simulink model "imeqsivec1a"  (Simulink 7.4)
settings: Solver=ode45  StartTime=0.0  StopTime=1  MaxStep=1e-3  RelTol=1e-3
libraries: simulink x1

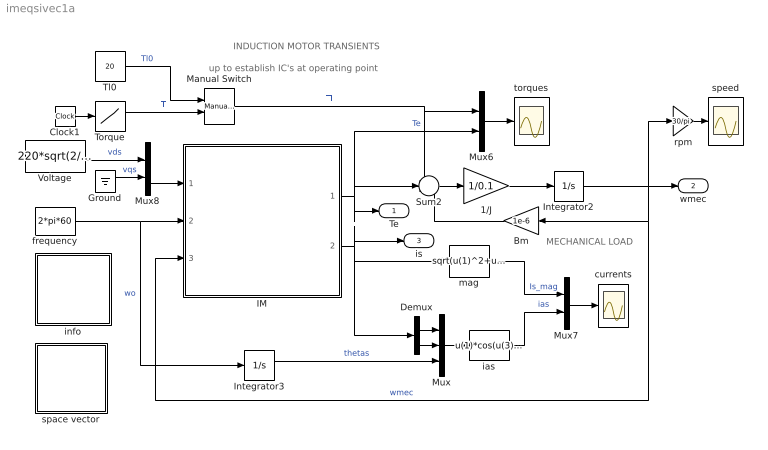
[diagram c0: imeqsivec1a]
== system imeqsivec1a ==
  note: INDUCTION MOTOR TRANSIENTS
  note: MECHANICAL LOAD
  note: up to establish IC's at operating point
  1/J : Gain  Gain=1/0.1  ParameterDataType=sfix(16)  ParameterScaling=2^0  OutDataType=sfix(16)  OutScaling=2^0
  Bm : Gain  Gain=1e-6  ParameterDataType=sfix(16)  ParameterScaling=2^0  OutDataType=sfix(16)  OutScaling=2^0
  Clock1 : Clock
  Demux : Demux  Outputs=2
  Ground : Ground
  IM : Subsystem  mask(Inductionmachine){Rs=0.531, Rr=0.408, Lsl=0.0025, Lrl=0.0025, Lm=0.085, wo=2*pi*60, p=4}
      mask prompts: Rs "Stator resistance [ohm]"; Rr "Rotor resistance [ohm]"; Lsl "Stator leakage inductance  [H]"; Lrl "Rotor leakage inductance [H]"; Lm "Magnetizing inductance [H]"; wo "Base frequency [rad/s]"; p "Number of poles"
      mask help: Space vector model of the induction machine in a general frame k. SI units
  Integrator2 : Integrator  InitialCondition=180
  Integrator3 : Integrator
  Manual Switch : simulink/Signal Routing/Manual Switch  SystemSampleTime=-1  sw=0  action=0  varsize=off
  Mux : Mux  Inputs=3
  Mux6 : Mux  Inputs=2
  Mux7 : Mux  Inputs=2
  Mux8 : Mux  Inputs=2
  Sum2 : Sum  Inputs=-+-  OutDataType=sfix(16)  OutScaling=2^0
  Tl0 : Constant  Value=20  OutDataType=sfix(16)  OutScaling=2^0
  Torque : Lookup  InputValues=[0 0.2 0.2 0.5 0.5 1]  Table=[20 20 10 10 20 20]  OutDataType=sfix(16)  OutScaling=2^0
  Voltage : Constant  Value=220*sqrt(2/3)  OutDataType=sfix(16)  OutScaling=2^0
  currents : Scope
  frequency : Constant  Value=2*pi*60  OutDataType=sfix(16)  OutScaling=2^0
  ias : Fcn  Expr=u(1)*cos(u(3))-u(2)*sin(u(3))
  info : Subsystem
  mag : Fcn  Expr=sqrt(u(1)^2+u(2)^2)
  rpm : Gain  Gain=30/pi  ParameterDataType=sfix(16)  ParameterScaling=2^0  OutDataType=sfix(16)  OutScaling=2^0
  space vector : Subsystem
  speed : Scope
  torques : Scope
  Te : Outport
  wmec : Outport  Port=2
  is : Outport  Port=3
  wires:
  mag/1 -> Mux7/1  "Is_mag"
  Sum2/1 -> 1/J/1
  1/J/1 -> Integrator2/1
  Mux8/1 -> IM/1(vs)
  Ground/1 -> Mux8/2  "vqs"
  IM/1(Te) -> Sum2/2, Te/1, Mux6/2  "Te"
  IM/2(is) -> is/1, Demux/1, mag/1
  Mux6/1 -> torques/1
  Bm/1 -> Sum2/3
  Mux7/1 -> currents/1
  Voltage/1 -> Mux8/1  "vds"
  frequency/1 -> Integrator3/1, IM/2(wk)  "wo"
  Demux/1 -> Mux/1
  Demux/2 -> Mux/2
  Mux/1 -> ias/1
  ias/1 -> Mux7/2  "ias"
  Integrator3/1 -> Mux/3  "thetas"
  Clock1/1 -> Torque/1
  Torque/1 -> Manual Switch/2  "Tl"
  Tl0/1 -> Manual Switch/1  "Tl0"
  Manual Switch/1 -> Mux6/1, Sum2/1  "Tl"
  Integrator2/1 -> wmec/1, IM/3(wmec), Bm/1, rpm/1  "wmec"
  rpm/1 -> speed/1

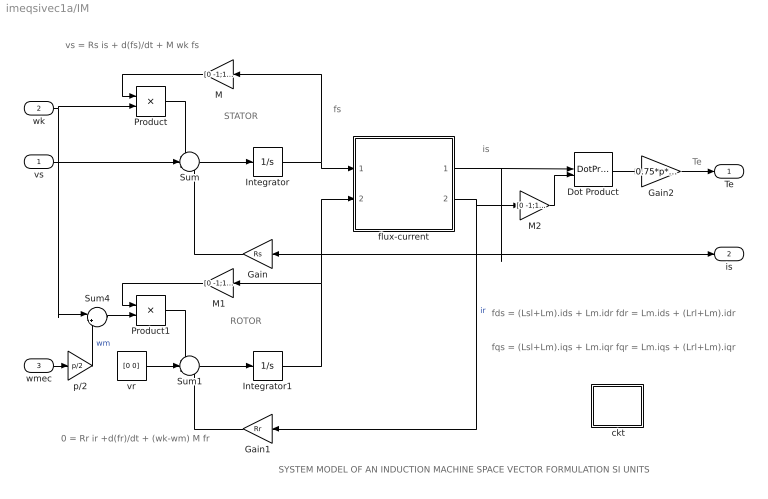
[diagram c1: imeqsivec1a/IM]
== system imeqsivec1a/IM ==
  note: ROTOR
  note: STATOR
  note: fs
  note: is
  note: Te
  note: SYSTEM MODEL OF AN INDUCTION MACHINE SPACE VECTOR FORMULATION SI UNITS
  note: vs = Rs is + d(fs)/dt + M wk fs
  note: 0 = Rr ir +d(fr)/dt + (wk-wm) M fr
  note: fds = (Lsl+Lm).ids + Lm.idr fdr = Lm.ids + (Lrl+Lm).idr
  note: fqs = (Lsl+Lm).iqs + Lm.iqr fqr = Lm.iqs + (Lrl+Lm).iqr
  vs : Inport  OutDataType=sfix(16)  OutScaling=2^0
  wk : Inport  Port=2  OutDataType=sfix(16)  OutScaling=2^0
  wmec : Inport  Port=3  OutDataType=sfix(16)  OutScaling=2^0
  " ckt" : Subsystem
  Dot Product : DotProduct  OutDataType=fixdt(1, 16)  OutScaling=2^-10
  Gain : Gain  Gain=Rs  ParameterDataType=sfix(16)  ParameterScaling=2^0  OutDataType=sfix(16)  OutScaling=2^0
  Gain1 : Gain  Gain=Rr  ParameterDataType=sfix(16)  ParameterScaling=2^0  OutDataType=sfix(16)  OutScaling=2^0
  Gain2 : Gain  Gain=0.75*p*Lm  ParameterDataType=sfix(16)  ParameterScaling=2^0  OutDataType=sfix(16)  OutScaling=2^0
  Integrator : Integrator  InitialCondition=[0 0]
  Integrator1 : Integrator  InitialCondition=[0 0]
  M : Gain  Gain=[0 -1;1 0]  Multiplication=Matrix(K*u)  ParameterDataType=sfix(16)  ParameterScaling=2^0  OutDataType=sfix(16)  OutScaling=2^0
  M1 : Gain  Gain=[0 -1;1 0]  Multiplication=Matrix(K*u)  ParameterDataType=sfix(16)  ParameterScaling=2^0  OutDataType=sfix(16)  OutScaling=2^0
  M2 : Gain  Gain=[0 -1;1 0]  Multiplication=Matrix(K*u)  ParameterDataType=sfix(16)  ParameterScaling=2^0  OutDataType=sfix(16)  OutScaling=2^0
  Product : Product  OutDataType=sfix(16)  OutScaling=2^0
  Product1 : Product  OutDataType=sfix(16)  OutScaling=2^0
  Sum : Sum  Inputs=-+-  OutDataType=sfix(16)  OutScaling=2^0
  Sum1 : Sum  Inputs=-+-  OutDataType=sfix(16)  OutScaling=2^0
  Sum4 : Sum  Inputs=|+-  OutDataType=sfix(16)  OutScaling=2^0
  flux-current : Subsystem
  p/2 : Gain  Gain=p/2  ParameterDataType=sfix(16)  ParameterScaling=2^0  OutDataType=sfix(16)  OutScaling=2^0
  vr : Constant  Value=[0 0]  OutDataType=sfix(16)  OutScaling=2^0
  Te : Outport
  is : Outport  Port=2
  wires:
  Gain/1 -> Sum/3
  vr/1 -> Sum1/2
  Gain1/1 -> Sum1/3
  Integrator/1 -> flux-current/1(fs), M/1
  Integrator1/1 -> flux-current/2(fr), M1/1
  Product1/1 -> Sum1/1
  M1/1 -> Product1/1
  Product/1 -> Sum/1
  M/1 -> Product/1
  Sum4/1 -> Product1/2
  vs/1 -> Sum/2
  wk/1 -> Product/2, Sum4/1
  Sum1/1 -> Integrator1/1
  Sum/1 -> Integrator/1
  flux-current/1(is) -> Gain/1, is/1, Dot Product/1
  flux-current/2(ir) -> Gain1/1, M2/1  "ir"
  Dot Product/1 -> Gain2/1
  Gain2/1 -> Te/1
  wmec/1 -> p/2/1
  p/2/1 -> Sum4/2  "wm"
  M2/1 -> Dot Product/2

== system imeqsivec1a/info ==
  note: Running of an induction motor under balanced sinusoidal excitation
  note: This demonstration illustrates the steady-state running of an induction motor at a specified load followed by sudden step changes in load. First establish the operating point IC's by connecting the manual switch to the up position and saving to workspace the simulation parameters defined as "Final state" ic; Run the simulation for a long enough time to reach a steady-state condition (dc). Then switch down and load from workspace the previously computed ic as "Initial state". Finally rerun the simulation. To modify the machine parameters, double click the induction motor block.

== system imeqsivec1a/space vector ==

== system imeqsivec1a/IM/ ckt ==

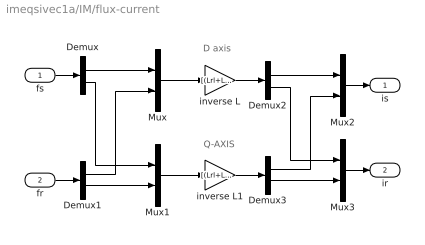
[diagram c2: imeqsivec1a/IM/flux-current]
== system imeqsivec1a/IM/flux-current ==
  note: D axis
  note: Q-AXIS
  fs : Inport  OutDataType=sfix(16)  OutScaling=2^0
  fr : Inport  Port=2  OutDataType=sfix(16)  OutScaling=2^0
  Demux{,1..3} (4 alike) : Demux  Outputs=2
  Mux{,1..3} (4 alike) : Mux  Inputs=2
  inverse L : Gain  Gain=[(Lrl+Lm) -Lm;-Lm (Lsl+Lm)]/(Lsl*Lrl+Lsl*Lm+Lrl*Lm)  Multiplication=Matrix(K*u)  ParameterDataType=sfix(16)  ParameterScaling=2^0  OutDataType=sfix(16)  OutScaling=2^0
  inverse L1 : Gain  Gain=[(Lrl+Lm) -Lm;-Lm (Lsl+Lm)]/(Lsl*Lrl+Lsl*Lm+Lrl*Lm)  Multiplication=Matrix(K*u)  ParameterDataType=sfix(16)  ParameterScaling=2^0  OutDataType=sfix(16)  OutScaling=2^0
  is : Outport
  ir : Outport  Port=2
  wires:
  Demux/1 -> Mux/1
  Mux/1 -> inverse L/1
  inverse L/1 -> Demux2/1
  Demux2/1 -> Mux2/1
  fs/1 -> Demux/1
  Mux2/1 -> is/1
  Demux1/1 -> Mux/2
  Demux1/2 -> Mux1/2
  Demux/2 -> Mux1/1
  Mux1/1 -> inverse L1/1
  inverse L1/1 -> Demux3/1
  Demux3/2 -> Mux3/2
  Demux2/2 -> Mux3/1
  Demux3/1 -> Mux2/2
  Mux3/1 -> ir/1
  fr/1 -> Demux1/1
